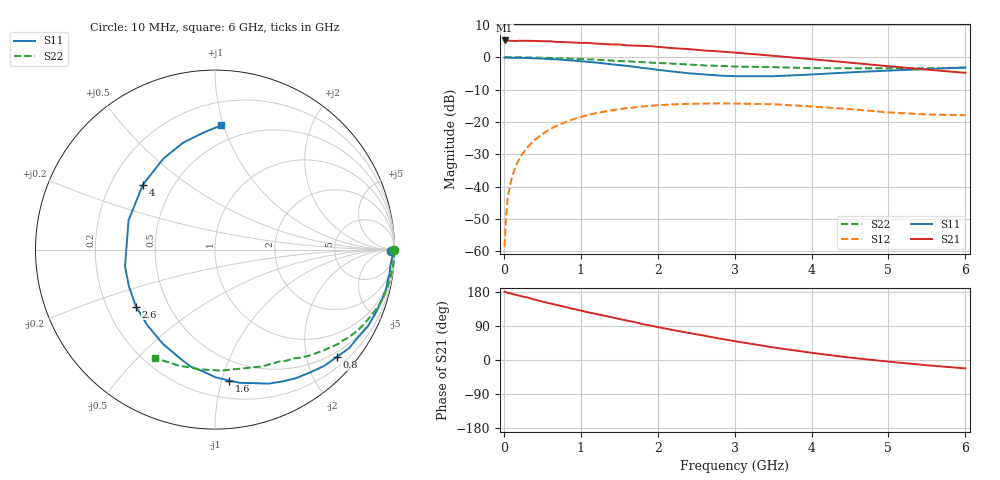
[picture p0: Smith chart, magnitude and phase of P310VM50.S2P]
! SIEMENS Small Signal Semiconductors
! BFP181
! Si NPN RF Bipolar Junction Transistor in SOT143
! VCE = 10 V  IC = 0.5 mA
! Common Emitter S-Parameters:  March  1996
# GHz  S  MA  R  50
!  f  S11  S21  S12  S22
! GHz  MAG  ANG  MAG  ANG  MAG  ANG  MAG  ANG
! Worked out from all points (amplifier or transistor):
!   36 points, 10 MHz to 6 GHz, reference 50 ohm
!   highest |S21| = 5.2 dB at 10 MHz (marker M1)
!   |S21| within 3 dB of that: start of sweep to 2.556 GHz
!   unconditionally stable (mu >= 1): 3.839 GHz to end of sweep
!   at 250 MHz: K = 0.08, MSG = 17.3 dB, |S12| = -29.6 dB
!   at 1.4 GHz: K = 0.41, MSG = 10.2 dB, |S12| = -16.4 dB
!   at 6 GHz: K = 1.42, MAG = 2.7 dB, |S12| = -17.9 dB
!   S11 on the Smith chart (normalised r, x): 10 MHz: open; 800 MHz: 0.39, -2.59; 1.6 GHz: 0.33, -1.06; 2.6 GHz: 0.32, -0.29; 4 GHz: 0.34, +0.35; 6 GHz: 0.37, +0.98
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0.01  0.9833 -0.6  1.817 179.8  0.0012 80.2  0.9988 -0.2
0.02  0.9928 -1.1  1.815 179.5  0.0024 81.3  0.9968 -0.5
0.05  0.9885 -2.5  1.807 177.5  0.0068 91.1  0.9979 -1.3
0.1  0.9814 -5.3  1.794 175.0  0.0132 84.5  0.9989 -2.6
0.15  0.9812 -8.0  1.785 172.3  0.0201 83.9  0.9958 -3.9
0.2  0.9775 -10.3  1.799 169.8  0.0268 81.5  0.996 -5.1
0.3  0.9719 -15.9  1.797 165.3  0.0398 78.5  0.9919 -7.8
0.4  0.9636 -20.8  1.787 159.4  0.0526 75.2  0.9877 -10.3
0.6  0.9347 -31.4  1.766 149.5  0.0773 67.4  0.9748 -15.4
0.8  0.9041 -41.5  1.713 139.9  0.0993 60.3  0.9576 -20.1
1.1  0.8471 -57.6  1.665 125.7  0.1284 49.8  0.9256 -27.0
1.5  0.7559 -79.2  1.572 108.3  0.1569 37.4  0.8748 -35.3
1.6  0.7343 -83.7  1.529 104.0  0.1632 34.8  0.8659 -37.1
1.9  0.665 -101.9  1.483 91.1  0.1772 26.4  0.827 -42.7
2.2  0.5999 -119.0  1.381 78.9  0.1869 19.0  0.7942 -47.7
2.6  0.5427 -144.2  1.272 64.4  0.192 10.2  0.7487 -54.0
3  0.5096 -169.5  1.18 49.7  0.192 1.7  0.7188 -60.3
3.5  0.5088 161.2  1.053 33.3  0.1881 -6.9  0.7018 -68.1
4  0.5409 137.9  0.933 19.0  0.1731 -13.4  0.6793 -77.2
4.5  0.5831 119.5  0.824 6.3  0.1577 -18.3  0.675 -87.1
5.5  0.6553 95.6  0.644 -13.9  0.1304 -16.7  0.6777 -107.9
6  0.6937 87.1  0.574 -22.2  0.1272 -13.1  0.6892 -118.8
